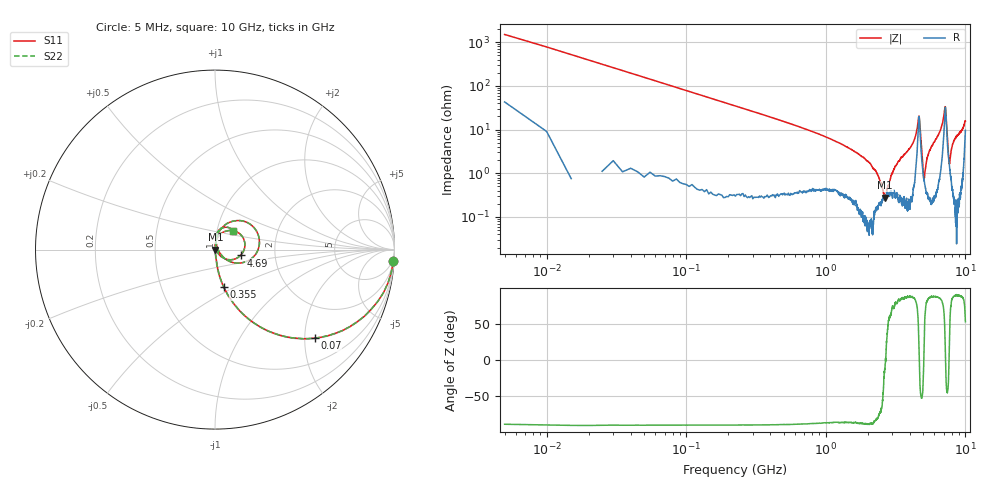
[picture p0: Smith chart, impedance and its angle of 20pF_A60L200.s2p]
! Amotech Co.,Ltd.
! http://www.amotech.co.kr/
! Part Number: A60L200
! These Parameters are Measured in Series Mode Connection
! Operation Temp=25[degC], DC Bias Voltage=0[V]
! Freq. Start=5[MHz] Stop=10[GHz], 2000[Steps]
! Date: Monday, July 14, 2020, 09:37:11
# GHZ S RI R 50.000000
!Freq.(Hz) S11(Real) S11(Imag) S21(Real) S21(Imag) S12(Real) S12(Imag) S22(Real) S22(Imag)
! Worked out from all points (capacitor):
!   2000 points, 5 MHz to 10 GHz, reference 50 ohm
!   read as one part in series: C = 20.3 pF near 55 MHz
!   lowest |Z| = 275 mohm at 2.665 GHz (marker M1)
!   series resonance near 2.678 GHz, so ESL is about 170 pH
!   S11 on the Smith chart (normalised r, x): 5 MHz: 2, -30; 70 MHz: 1.02, -2.24; 355 MHz: 1.01, -0.44; 4.69 GHz: 1.33, -0.09; 10 GHz: 1.19, +0.25
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0.005  0.9937 -0.0661  0.0063 0.0661  0.0063 0.0661  0.9937 -0.0661
0.07  0.5563 -0.4931  0.4437 0.4931  0.4437 0.4931  0.5563 -0.4931
0.17  0.1775 -0.3784  0.8225 0.3784  0.8225 0.3784  0.1775 -0.3784
0.355  0.0483 -0.208  0.9517 0.208  0.9517 0.208  0.0483 -0.208
1.675  0.00276 -0.029  0.9972 0.029  0.9972 0.029  0.00276 -0.029
2.285  0.0015 -0.0111  0.9985 0.0111  0.9985 0.0111  0.0015 -0.0111
2.665  0.00273 -0.000235  0.9973 0.000235  0.9973 0.000235  0.00273 -0.000235
2.975  0.0034 0.00903  0.9966 -0.00903  0.9966 -0.00903  0.0034 0.00903
3.34  0.00294 0.019  0.9971 -0.019  0.9971 -0.019  0.00294 0.019
4.205  0.00609 0.0479  0.9939 -0.0479  0.9939 -0.0479  0.00609 0.0479
4.615  0.1324 0.0924  0.8676 -0.0924  0.8676 -0.0924  0.1324 0.0924
4.69  0.1422 -0.0327  0.8578 0.0327  0.8578 0.0327  0.1422 -0.0327
5.005  0.00827 -0.00348  0.9917 0.00348  0.9917 0.00348  0.00827 -0.00348
5.07  0.00677 0.00353  0.9932 -0.00353  0.9932 -0.00353  0.00677 0.00353
5.295  0.00383 0.0203  0.9962 -0.0203  0.9962 -0.0203  0.00383 0.0203
5.515  0.00366 0.0316  0.9963 -0.0316  0.9963 -0.0316  0.00366 0.0316
6.67  0.0221 0.0988  0.9779 -0.0988  0.9779 -0.0988  0.0221 0.0988
7.055  0.139 0.1617  0.861 -0.1617  0.861 -0.1617  0.139 0.1617
7.185  0.247 0.0287  0.753 -0.0287  0.753 -0.0287  0.247 0.0287
7.675  0.0152 0.00578  0.9848 -0.00578  0.9848 -0.00578  0.0152 0.00578
8.335  0.00524 0.0573  0.9948 -0.0573  0.9948 -0.0573  0.00524 0.0573
10  0.0993 0.1029  0.9007 -0.1029  0.9007 -0.1029  0.0993 0.1029
